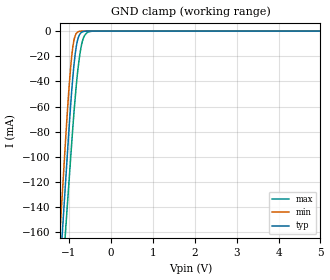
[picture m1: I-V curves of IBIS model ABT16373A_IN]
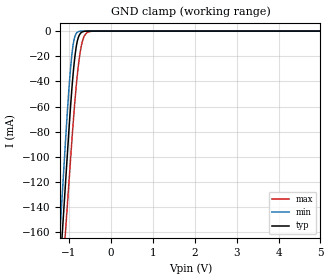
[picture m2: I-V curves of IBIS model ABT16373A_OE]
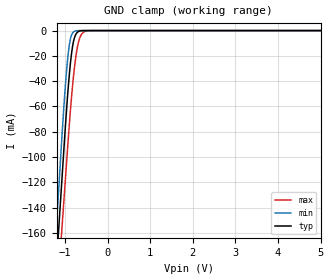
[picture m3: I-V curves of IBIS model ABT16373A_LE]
| TEXAS INSTRUMENTS INCORPORATED
| Standard Linear and Logic Group
| IBIS Model of SN74ABT16373A
| 16-BIT TRANSPARENT D-TYPE LATCHES WITH 3-STATE OUTPUTS
| This file contains package information for the following:
|   TSSOP 48-pin (DGG) package as [Component] ABT16373A_DGG
|   SSOP 48-pin (DL) package as [Component] ABT16373A_DL
| This device can be powered at the following Vccs:
|   5 volt Vcc
| This file provides unique models under the [Model Selector] for each Vcc.
| For operation at a specific Vcc, select the appropriate model after each
| [Model Selector] keyword.
[IBIS Ver]   3.2
[Comment char]  |_char
[File Name]   sn74abt16373a.ibs
[File Rev]   1.1 | b_die
[Date]   June 19, 2002
[Source]   Data created from TI-SPICE simulations at TI-SLL.
[Notes]   The following is an IBIS list for the SN74ABT16373A.
   Please contact sllibis@ti.com with questions and
   comments concerning SLL IBIS models.
   This IBIS model is created from a BA (back annotated netlist).
   - FILE REV HISTORY
   - 1.1 Release IBIS file on 12/21/05
   - Non-Convergence in the following files:
   gc_ABT16373A_IN, extrapolated from 0.5 V plus
   pc_ABT16373A_IN, extrapolated from 1.38 V plus
   - The device has series-clamp diode at the output which causes
   non-monotonic behavior
   - C_comp values are taken at a different test condition
   than the Ci in data sheet.
   - C_comp values are taken at a different test condition
   than the Co in data sheet.
   - Power clamp data has been deleted since there is no
   power clamp diode in the device.
   - End point warning due to AC and DC mismatch.
[Disclaimer] Property of Texas Instruments Incorporated. Unauthorized
   reproduction and/or distribution is strictly prohibited.
   This product is protected under copyright law.
   Created 2002, (C) Copyright 2002, Texas Instruments
   Incorporated, All Rights Reserved
   UNLESS THERE IS A SIGNED, WRITTEN AGREEMENT TO THE
   CONTRARY, TEXAS INSTRUMENTS (TI) IS PROVIDING THE IBIS
   MODELS  AND WITHOUT ANY WARRANTY, EXPRESSED OR
   IMPLIED. TI assumes no liability for:
   1) the accuracy of the IBIS models provided to your
   company;
   2) the proper functioning of these IBIS Models in your
   design or for any resulting applications; or
   3) infringement of patents, copyrights or intellectual
   property rights resulting from your use of these IBIS
   models.
   TI provides IBIS Models as a service to our customers.
   You and your company shall not distribute, sell or give
   these models to anyone else without prior written
   permission from TI.
   TI reserves the right to make changes to our products or
   to discontinue any semiconductor product or service
   without notice, and advises our customers to obtain the
   latest version of relevant information to verify, before
   placing orders, that the information being relied on is
   current.
   Please be aware that your receipt and use of the IBIS
   information provided shall serve as acceptance of these
   terms and conditions. If you do not accept these terms,
   you should return or destroy the IBIS models and any
   other accompanying information immediately.
| Component ABT16373A_DGG 48-pin TSSOP
[Component]   ABT16373A_DGG
[Manufacturer]  Texas Instruments, Inc.
[Package]
|   typ   min   max
R_pkg   4.400e-02   3.800e-02   5.100e-02
L_pkg   3.019e-09   2.486e-09   4.099e-09
C_pkg   5.070e-13   3.340e-13   8.090e-13
[Pin]   signal_name   model_name   R_pin   L_pin   C_pin
1   1NOE   ABT16373A_OE   4.100e-02   4.017e-09   7.590e-13
2   1Q1   ABT16373A_OUT   4.200e-02   3.737e-09   7.920e-13
3   1Q2   ABT16373A_OUT   4.200e-02   3.480e-09   6.610e-13
4   GND   GND   3.800e-02   3.131e-09   5.750e-13
5   1Q3   ABT16373A_OUT   4.700e-02   3.122e-09   5.660e-13
6   1Q4   ABT16373A_OUT   4.300e-02   2.948e-09   5.040e-13
7   VCC   POWER   4.500e-02   2.845e-09   3.970e-13
8   1Q5   ABT16373A_OUT   4.900e-02   2.835e-09   3.940e-13
9   1Q6   ABT16373A_OUT   4.800e-02   2.715e-09   3.780e-13
10   GND   GND   5.000e-02   2.664e-09   3.630e-13
11   1Q7   ABT16373A_OUT   5.000e-02   2.585e-09   3.480e-13
12   1Q8   ABT16373A_OUT   4.900e-02   2.550e-09   3.370e-13
13   2Q1   ABT16373A_OUT   4.900e-02   2.541e-09   3.360e-13
14   2Q2   ABT16373A_OUT   5.000e-02   2.574e-09   3.480e-13
15   GND   GND   4.900e-02   2.618e-09   3.590e-13
16   2Q3   ABT16373A_OUT   4.600e-02   2.671e-09   3.750e-13
17   2Q4   ABT16373A_OUT   4.500e-02   2.754e-09   3.890e-13
18   VCC   POWER   4.400e-02   2.823e-09   4.500e-13
19   2Q5   ABT16373A_OUT   4.200e-02   2.968e-09   5.030e-13
20   2Q6   ABT16373A_OUT   5.100e-02   3.108e-09   5.350e-13
21   GND   GND   4.200e-02   3.175e-09   5.870e-13
22   2Q7   ABT16373A_OUT   4.100e-02   3.449e-09   6.780e-13
23   2Q8   ABT16373A_OUT   4.400e-02   3.766e-09   8.040e-13
24   2NOE   ABT16373A_OE   4.300e-02   4.065e-09   7.610e-13
25   2LE   ABT16373A_LE   4.100e-02   3.994e-09   7.570e-13
26   2D8   ABT16373A_IN   3.900e-02   3.649e-09   7.890e-13
27   2D7   ABT16373A_IN   3.800e-02   3.362e-09   6.600e-13
28   GND   GND   3.800e-02   3.082e-09   5.740e-13
29   2D6   ABT16373A_IN   4.400e-02   2.990e-09   5.220e-13
30   2D5   ABT16373A_IN   4.100e-02   2.917e-09   4.950e-13
31   VCC   POWER   4.300e-02   2.820e-09   4.480e-13
32   2D4   ABT16373A_IN   4.300e-02   2.699e-09   3.850e-13
33   2D3   ABT16373A_IN   4.500e-02   2.628e-09   3.720e-13
34   GND   GND   4.600e-02   2.556e-09   3.560e-13
35   2D2   ABT16373A_IN   4.600e-02   2.495e-09   3.440e-13
36   2D1   ABT16373A_IN   4.700e-02   2.487e-09   3.340e-13
37   1D8   ABT16373A_IN   4.700e-02   2.490e-09   3.350e-13
38   1D7   ABT16373A_IN   4.600e-02   2.486e-09   3.430e-13
39   GND   GND   4.500e-02   2.566e-09   3.560e-13
40   1D6   ABT16373A_IN   4.400e-02   2.639e-09   3.740e-13
41   1D5   ABT16373A_IN   4.300e-02   2.701e-09   3.860e-13
42   VCC   POWER   4.300e-02   2.817e-09   4.500e-13
43   1D4   ABT16373A_IN   4.100e-02   2.935e-09   5.010e-13
44   1D3   ABT16373A_IN   4.700e-02   3.035e-09   5.290e-13
45   GND   GND   4.300e-02   3.171e-09   5.890e-13
46   1D2   ABT16373A_IN   4.000e-02   3.415e-09   6.820e-13
47   1D1   ABT16373A_IN   4.300e-02   3.741e-09   8.090e-13
48   1LE   ABT16373A_LE   4.400e-02   4.099e-09   7.640e-13
| Component ABT16373A_DL 48-pin SSOP
[Component]   ABT16373A_DL
[Manufacturer]  Texas Instruments, Inc.
[Package]
|   typ   min   max
R_pkg   4.800e-02   3.800e-02   5.300e-02
L_pkg   6.046e-09   5.084e-09   7.968e-09
C_pkg   8.130e-13   5.690e-13   1.157e-12
[Pin]   signal_name   model_name   R_pin   L_pin   C_pin
1   1NOE   ABT16373A_OE   4.600e-02   7.968e-09   1.017e-12
2   1Q1   ABT16373A_OUT   4.400e-02   7.299e-09   1.157e-12
3   1Q2   ABT16373A_OUT   4.300e-02   6.765e-09   1.058e-12
4   GND   GND   4.100e-02   6.269e-09   9.330e-13
5   1Q3   ABT16373A_OUT   3.800e-02   5.856e-09   8.290e-13
6   1Q4   ABT16373A_OUT   4.600e-02   5.802e-09   7.900e-13
7   VCC   POWER   5.000e-02   5.656e-09   7.380e-13
8   1Q5   ABT16373A_OUT   5.300e-02   5.500e-09   6.430e-13
9   1Q6   ABT16373A_OUT   5.200e-02   5.304e-09   6.060e-13
10   GND   GND   5.300e-02   5.189e-09   5.830e-13
11   1Q7   ABT16373A_OUT   5.100e-02   5.084e-09   5.690e-13
12   1Q8   ABT16373A_OUT   5.300e-02   5.862e-09   8.330e-13
13   2Q1   ABT16373A_OUT   5.300e-02   5.862e-09   8.330e-13
14   2Q2   ABT16373A_OUT   5.100e-02   5.084e-09   5.690e-13
15   GND   GND   5.300e-02   5.189e-09   5.830e-13
16   2Q3   ABT16373A_OUT   5.200e-02   5.304e-09   6.060e-13
17   2Q4   ABT16373A_OUT   5.300e-02   5.500e-09   6.430e-13
18   VCC   POWER   5.000e-02   5.656e-09   7.380e-13
19   2Q5   ABT16373A_OUT   4.600e-02   5.802e-09   7.900e-13
20   2Q6   ABT16373A_OUT   3.800e-02   5.856e-09   8.290e-13
21   GND   GND   4.100e-02   6.269e-09   9.330e-13
22   2Q7   ABT16373A_OUT   4.300e-02   6.765e-09   1.058e-12
23   2Q8   ABT16373A_OUT   4.400e-02   7.299e-09   1.157e-12
24   2NOE   ABT16373A_OE   4.600e-02   7.968e-09   1.017e-12
25   2LE   ABT16373A_LE   4.600e-02   7.968e-09   1.017e-12
26   2D8   ABT16373A_IN   4.400e-02   7.299e-09   1.157e-12
27   2D7   ABT16373A_IN   4.300e-02   6.765e-09   1.058e-12
28   GND   GND   4.100e-02   6.269e-09   9.330e-13
29   2D6   ABT16373A_IN   3.800e-02   5.856e-09   8.290e-13
30   2D5   ABT16373A_IN   4.600e-02   5.802e-09   7.900e-13
31   VCC   POWER   5.000e-02   5.656e-09   7.380e-13
32   2D4   ABT16373A_IN   5.300e-02   5.500e-09   6.430e-13
33   2D3   ABT16373A_IN   5.200e-02   5.304e-09   6.060e-13
34   GND   GND   5.300e-02   5.189e-09   5.830e-13
35   2D2   ABT16373A_IN   5.100e-02   5.084e-09   5.690e-13
36   2D1   ABT16373A_IN   5.300e-02   5.862e-09   8.330e-13
37   1D8   ABT16373A_IN   5.300e-02   5.862e-09   8.330e-13
38   1D7   ABT16373A_IN   5.100e-02   5.084e-09   5.690e-13
39   GND   GND   5.300e-02   5.189e-09   5.830e-13
40   1D6   ABT16373A_IN   5.200e-02   5.304e-09   6.060e-13
41   1D5   ABT16373A_IN   5.300e-02   5.500e-09   6.430e-13
42   VCC   POWER   5.000e-02   5.656e-09   7.380e-13
43   1D4   ABT16373A_IN   4.600e-02   5.802e-09   7.900e-13
44   1D3   ABT16373A_IN   3.800e-02   5.856e-09   8.290e-13
45   GND   GND   4.100e-02   6.269e-09   9.330e-13
46   1D2   ABT16373A_IN   4.300e-02   6.765e-09   1.058e-12
47   1D1   ABT16373A_IN   4.400e-02   7.299e-09   1.157e-12
48   1LE   ABT16373A_LE   4.600e-02   7.967e-09   1.017e-12
| Models and submodels in the file (4): ABT16373A_IN (Input), ABT16373A_OE (Input), ABT16373A_LE (Input), ABT16373A_OUT (3-state)
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[Model]   ABT16373A_IN
Model_type  Input
Vinl=0.8
Vinh=2.0
| variable   typ   min   max
C_comp   3.09pF   2.52pF   4.56pF
[Temperature Range]   40   -40   100
| Ambient temperature   25   -40   85
[Voltage range]   5   4.5   5.5
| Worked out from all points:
|   GND clamp passes 1 mA (typ) near -0.70 V on its own axis
[GND Clamp]
| ABT16373A_IN
|   Voltage   I(typ)   I(min)   I(max)
-5V       -2.153A    -2.252A    -2.029A
-1.27V    -219.8mA   -192.6mA   -250.3mA
-1.165V   -165.3mA   -134.6mA   -200.3mA
-1.075V   -118.7mA   -84.94mA   -157.4mA
-1V       -79.84mA   -47.06mA   -121.6mA
-925mV    -44.85mA   -17.94mA   -85.91mA
-850mV    -18.77mA   -3.745mA   -53.68mA
-775mV    -5.229mA   -456uA     -28.13mA
-725mV    -1.881mA   -65.53uA   -15.89mA
-650mV    -301.3uA   -1.883uA   -5.398mA
-475mV    -495.5nA   -657.9pA   -218.9uA
5V        60.29pA    64.86pA    153.2pA
[Model]   ABT16373A_OE
Model_type  Input
Vinl=0.8
Vinh=2.0
| variable   typ   min   max
C_comp   2.97pF   2.42pF   4.54pF
[Temperature Range]   40   -40   100
| Ambient temperature   25   -40   85
[Voltage range]   5   4.5   5.5
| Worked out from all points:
|   GND clamp passes 1 mA (typ) near -0.70 V on its own axis
[GND Clamp]
| ABT16373A_OE
|   Voltage   I(typ)   I(min)   I(max)
-5V       -2.153A    -2.252A    -2.029A
-1.27V    -219.8mA   -192.6mA   -250.3mA
-1.165V   -165.3mA   -134.6mA   -200.3mA
-1.075V   -118.7mA   -84.94mA   -157.4mA
-1V       -79.84mA   -47.06mA   -121.6mA
-925mV    -44.85mA   -17.94mA   -85.91mA
-850mV    -18.77mA   -3.745mA   -53.68mA
-775mV    -5.229mA   -456uA     -28.13mA
-725mV    -1.881mA   -65.53uA   -15.89mA
-650mV    -301.3uA   -1.883uA   -5.398mA
-475mV    -495.5nA   -657.9pA   -218.9uA
5V        60.29pA    64.86pA    153.2pA
[Model]   ABT16373A_LE
Model_type  Input
Vinl=0.8
Vinh=2.0
| variable   typ   min   max
C_comp   2.90pF   2.35pF   4.48pF
[Temperature Range]   40   -40   100
| Ambient temperature   25   -40   85
[Voltage range]   5   4.5   5.5
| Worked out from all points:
|   GND clamp passes 1 mA (typ) near -0.70 V on its own axis
[GND Clamp]
| ABT16373A_LE
|   Voltage   I(typ)   I(min)   I(max)
-5V       -2.153A    -2.252A    -2.029A
-1.27V    -219.8mA   -192.6mA   -250.3mA
-1.165V   -165.3mA   -134.6mA   -200.3mA
-1.075V   -118.7mA   -84.94mA   -157.4mA
-1V       -79.84mA   -47.06mA   -121.6mA
-925mV    -44.85mA   -17.94mA   -85.91mA
-850mV    -18.77mA   -3.745mA   -53.68mA
-775mV    -5.229mA   -456uA     -28.13mA
-725mV    -1.881mA   -65.53uA   -15.89mA
-650mV    -301.3uA   -1.883uA   -5.398mA
-475mV    -495.5nA   -657.9pA   -218.9uA
5V        60.29pA    64.86pA    153.2pA
